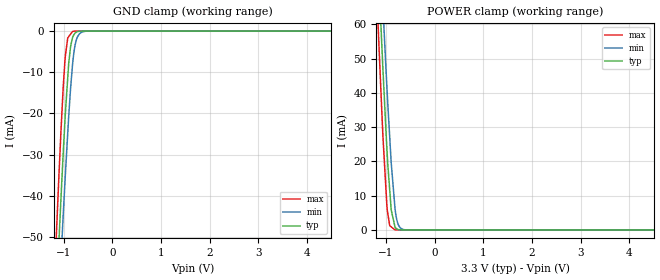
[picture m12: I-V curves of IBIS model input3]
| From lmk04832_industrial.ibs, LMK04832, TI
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|   input3 Model
[Model]   input3
Model_type   Input
Vinl = 0.4
Vinh = 1.2
|   typ   min   max
C_comp   0.3074pF   0.3004pF   0.3116pF
|  Where Nom  PVT is Nominal Process,   3.3V,  25C
|   Fast PVT is Strong Process,   3.45V, -40C
|   Slow PVT is Weak Process,   3.15V, 85C
[Model spec]
|subparameter
Vinl   0.400   0.370   0.430
Vinh   1.200   1.170   1.230
[Voltage Range]   3.3   3.15   3.45
|Junction Temperature
[Temperature Range]   25   85   -40
[Power Clamp Reference]   3.3   3.15   3.45
[GND Clamp Reference]   0   0   0
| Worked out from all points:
|   GND clamp passes 1 mA (typ) near -0.79 V on its own axis
|   POWER clamp passes 1 mA (typ) near -0.82 V on its own axis
[GND Clamp]
|   Voltage   I(typ)   I(min)   I(max)
-3.3V     -672.7mA   -647.6mA   -705.9mA
-1.171V   -70.78mA   -84.12mA   -55.94mA
-1.092V   -50.35mA   -64.75mA   -34.3mA
-1.053V   -40.5mA    -55.3mA    -24.2mA
-1.013V   -31.05mA   -46.07mA   -15.01mA
-963.6mV  -20.09mA   -34.97mA   -6.05mA
-894.3mV  -7.846mA   -20.72mA   -1.358mA
-854.7mV  -3.646mA   -13.73mA   -717.2uA
-815.1mV  -1.572mA   -8.086mA   -76.58uA
-726mV    -201.3uA   -1.759mA   -7.617uA
-547.8mV  -2.202uA   -43.96uA   -1.842uA
6.6V      0A         0A         0A
[POWER Clamp]
|   Voltage   I(typ)   I(min)   I(max)
-3.3V     834.6mA    808.2mA    869.6mA
-1.171V   80.82mA    97.59mA    62.56mA
-1.142V   71.19mA    88.42mA    52.41mA
-1.082V   52.45mA    70.41mA    33mA
-1.063V   46.4mA     64.53mA    26.94mA
-973.5mV  21.42mA    39.24mA    5.581mA
-924mV    11.49mA    26.9mA     1.225mA
-894.3mV  5.863mA    19.63mA    898.7uA
-815.1mV  819.3uA    6.103mA    27.6uA
-735.9mV  79.66uA    1.183mA    15uA
-597.3mV  13.17uA    39.94uA    13.58uA
6.6V      0A         0A         0A
